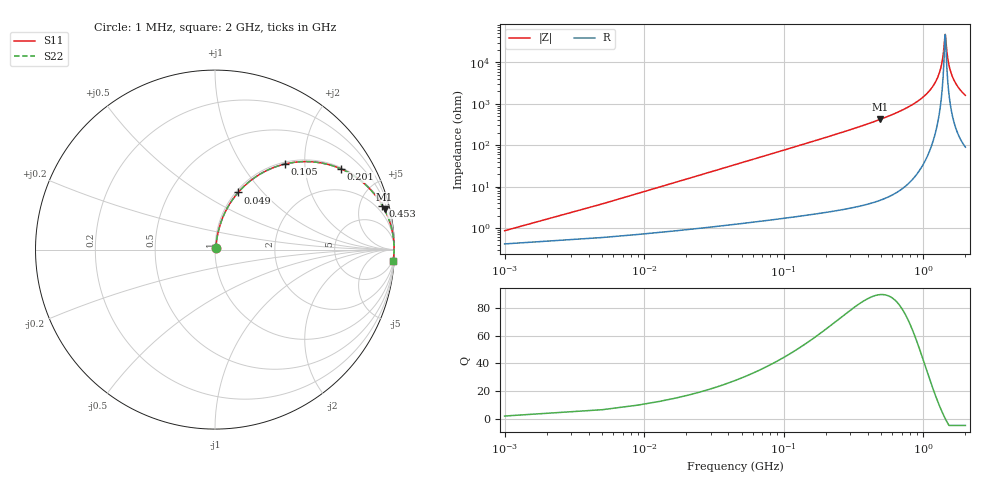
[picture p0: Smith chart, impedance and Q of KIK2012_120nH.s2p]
!version-2
!date-01.2022
!Series
# MHz S RI R 50
!Freq ReS11 ImS11 ReS21 ImS21 ReS12 ImS12 ReS22 ImS22
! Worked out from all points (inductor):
!   501 points, 1 MHz to 2 GHz, reference 50 ohm
!   read as one part in series: L = 120 nH near 9 MHz
!   highest Q = 89.7 at 493 MHz (marker M1), where L = 136 nH
!   self-resonance near 1.433 GHz
!   S11 on the Smith chart (normalised r, x): 1 MHz: 1.01, +0.02; 49 MHz: 1.03, +0.74; 105 MHz: 1.03, +1.59; 201 MHz: 1.05, +3.09; 453 MHz: 1.09, +7.59; 2 GHz: 3, -32
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1  0.00417 0.00748  0.9958 -0.00748  0.9958 -0.00748  0.00417 0.00748
13  0.0171 0.0956  0.9829 -0.0956  0.9829 -0.0956  0.0171 0.0956
17  0.0243 0.124  0.9757 -0.124  0.9757 -0.124  0.0243 0.124
29  0.0546 0.2047  0.9454 -0.2047  0.9454 -0.2047  0.0546 0.2047
49  0.1288 0.3182  0.8712 -0.3182  0.8712 -0.3182  0.1288 0.3182
105  0.3903 0.4769  0.6097 -0.4769  0.6097 -0.4769  0.3903 0.4769
201  0.7022 0.4496  0.2978 -0.4496  0.2978 -0.4496  0.7022 0.4496
337  0.8756 0.324  0.1244 -0.324  0.1244 -0.324  0.8756 0.324
453  0.9327 0.2451  0.0673 -0.2451  0.0673 -0.2451  0.9327 0.2451
493  0.9445 0.2234  0.0555 -0.2234  0.0555 -0.2234  0.9445 0.2234
669  0.9748 0.1509  0.0252 -0.1509  0.0252 -0.1509  0.9748 0.1509
1001  0.9938 0.0674  0.00618 -0.0674  0.00618 -0.0674  0.9938 0.0674
1209  0.9972 0.0316  0.00278 -0.0316  0.00278 -0.0316  0.9972 0.0316
1337  0.9979 0.0129  0.00212 -0.0129  0.00212 -0.0129  0.9979 0.0129
1381  0.9979 0.00692  0.00208 -0.00692  0.00208 -0.00692  0.9979 0.00692
1433  0.9979 0.000113  0.00212 -0.000113  0.00212 -0.000113  0.9979 0.000113
1445  0.9979 -0.00142  0.00214 0.00142  0.00214 0.00142  0.9979 -0.00142
1481  0.9978 -0.00595  0.00225 0.00595  0.00225 0.00595  0.9978 -0.00595
1521  0.9976 -0.0109  0.00241 0.0109  0.00241 0.0109  0.9976 -0.0109
1585  0.9972 -0.0185  0.00277 0.0185  0.00277 0.0185  0.9972 -0.0185
1669  0.9966 -0.028  0.00341 0.028  0.00341 0.028  0.9966 -0.028
2000  0.9926 -0.062  0.00739 0.062  0.00739 0.062  0.9926 -0.062
